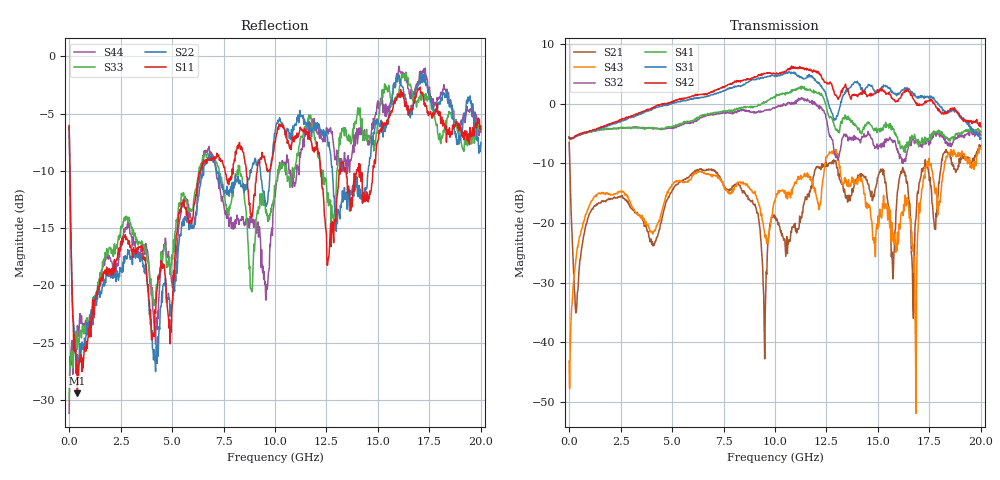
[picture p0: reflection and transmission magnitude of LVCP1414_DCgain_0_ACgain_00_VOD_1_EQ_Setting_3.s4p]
!Agilent Technologies,N5230A,MY46400459,A.07.50.48
!Agilent N5230A: A.07.50.48
!Date: Tuesday, April 17, 2012 18:26:47
!Correction: S11(Full 4 Port(1,2,3,4))
!S12(Full 4 Port(1,2,3,4))
!S13(Full 4 Port(1,2,3,4))
!S14(Full 4 Port(1,2,3,4))
!S21(Full 4 Port(1,2,3,4))
!S22(Full 4 Port(1,2,3,4))
!S23(Full 4 Port(1,2,3,4))
!S24(Full 4 Port(1,2,3,4))
!S31(Full 4 Port(1,2,3,4))
!S32(Full 4 Port(1,2,3,4))
!S33(Full 4 Port(1,2,3,4))
!S34(Full 4 Port(1,2,3,4))
!S41(Full 4 Port(1,2,3,4))
!S42(Full 4 Port(1,2,3,4))
!S43(Full 4 Port(1,2,3,4))
!S44(Full 4 Port(1,2,3,4))
!S4P File: Measurements: <S11,S12,S13,S14>,
!<S21,S22,S23,S24>,
!<S31,S32,S33,S34>,
!<S41,S42,S43,S44>:
# Hz S  dB  R 50
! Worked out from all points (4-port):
!   801 points, 300 kHz to 20 GHz, reference 50 ohm
!   strongest paths, dB at 300 kHz, 5 GHz, 10 GHz, 15 GHz, 20 GHz:
!     S42: -5.7, 0.4, 5.0, 2.3, -3.9
!     S31: -5.5, 0.1, 4.6, 2.0, -5.8
!     S41: -5.6, -3.8, 1.0, -4.3, -4.7
!     S32: -5.7, -4.1, -0.7, -7.6, -5.2
!     S43: -43.2, -13.5, -16.4, -18.8, -7.4
!     S21: -6.5, -14.6, -19.2, -12.3, -7.0
!   lowest |S11| = -29.4 dB at 400.3 MHz (marker M1), VSWR 1.07, Z = 53.1 + j1.56 ohm
!   |S11| at or under -10 dB: 37.54 MHz to 6.368 GHz (6.33 GHz wide, 198 % of centre); 12.22 GHz to 13.12 GHz (900.9 MHz wide, 7.11 % of centre); 14.14 GHz to 14.75 GHz (609.6 MHz wide, 4.22 % of centre)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
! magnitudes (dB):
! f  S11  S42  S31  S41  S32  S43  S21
! 300 kHz  -6.0  -5.7  -5.5  -5.6  -5.7  -43.2  -6.5
! 400.3 MHz  -29.4  -5.3  -5.2  -5.3  -5.3  -24.1  -31.7
! 10.03 GHz  -7.3  5.1  4.7  1.4  -0.6  -15.8  -19.0
! 12.88 GHz  -14.5  1.9  -2.8  -3.6  -8.1  -8.3  -9.6
! 16.8 GHz  -3.6  0.4  1.4  -5.5  -6.5  -34.7  -20.7
! 17.4 GHz  -4.9  0.5  1.3  -6.1  -6.1  -9.6  -10.2
! 20 GHz  -6.4  -3.9  -5.8  -4.7  -5.2  -7.4  -7.0
